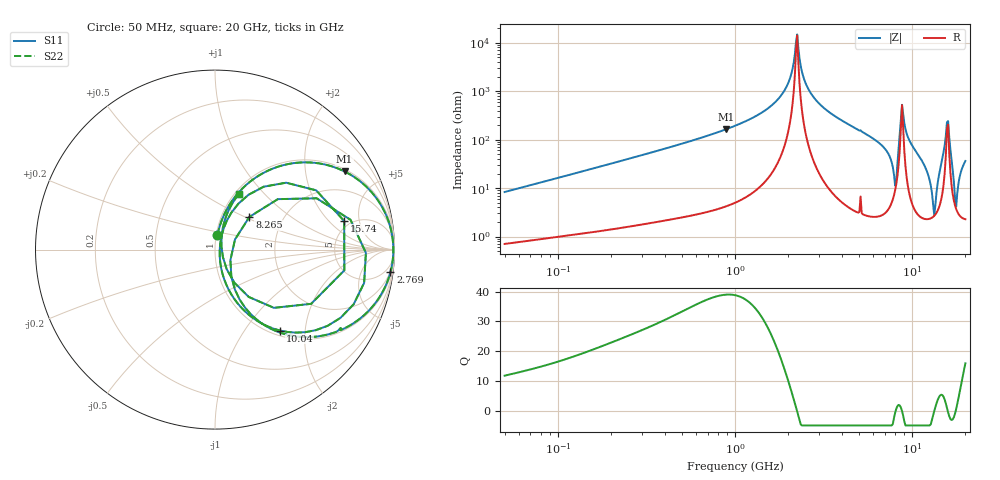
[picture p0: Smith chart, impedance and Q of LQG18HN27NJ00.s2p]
!Murata Part Number: LQG18HN27NJ00
!These Parameters are Measured in Series Mode Connection
!  o--[Z]--o
!Port1  Port2
!  o-------o
!Freq. Start=50[MHz] Stop=20[GHz], 401[Steps]
# Hz S RI R 50
!Freq.(Hz) S11(Real) S11(Imag) S21(Real) S21(Imag) S12(Real) S12(Imag) S22(Real) S22(Imag)
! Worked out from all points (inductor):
!   401 points, 50 MHz to 20 GHz, reference 50 ohm
!   read as one part in series: L = 26.1 nH near 51.52 MHz
!   highest Q = 39 at 887.1 MHz (marker M1), where L = 29.2 nH
!   self-resonance near 2.212 GHz
!   S11 on the Smith chart (normalised r, x): 50 MHz: 1.01, +0.17; 2.769 GHz: 2, -15; 8.265 GHz: 1.36, +0.53; 10.04 GHz: 1.09, -1.48; 15.74 GHz: 4.40, +3.07; 20 GHz: 1.05, +0.72
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5e7  0.0137 0.0811  0.9863 -0.0811  0.9863 -0.0811  0.0137 0.0811
1.364002e8  0.0559 0.2051  0.9441 -0.2051  0.9441 -0.2051  0.0559 0.2051
3.721004e8  0.2728 0.4288  0.7272 -0.4288  0.7272 -0.4288  0.2728 0.4288
8.870719e8  0.7217 0.4355  0.2783 -0.4355  0.2783 -0.4355  0.7217 0.4355
1e9  0.7827 0.3997  0.2173 -0.3997  0.2173 -0.3997  0.7827 0.3997
1.793498e9  0.9763 0.1272  0.0237 -0.1272  0.0237 -0.1272  0.9763 0.1272
2.021818e9  0.9898 0.0591  0.0102 -0.0591  0.0102 -0.0591  0.9898 0.0591
2.245319e9  0.9936 -0.00204  0.00638 0.00204  0.00638 0.00204  0.9936 -0.00204
2.728004e9  0.9795 -0.1178  0.0205 0.1178  0.0205 0.1178  0.9795 -0.1178
2.769174e9  0.9772 -0.1268  0.0228 0.1268  0.0228 0.1268  0.9772 -0.1268
7.442007e9  0.1972 -0.3576  0.8028 0.3576  0.8028 0.3576  0.1972 -0.3576
7.901521e9  0.0909 -0.1504  0.9091 0.1504  0.9091 0.1504  0.0909 -0.1504
8.264682e9  0.1922 0.1827  0.8078 -0.1827  0.8078 -0.1827  0.1922 0.1827
8.907419e9  0.831 -0.1852  0.169 0.1852  0.169 0.1852  0.831 -0.1852
1.004137e10  0.3632 -0.4512  0.6368 0.4512  0.6368 0.4512  0.3632 -0.4512
1.201863e10  0.0736 -0.2179  0.9264 0.2179  0.9264 0.2179  0.0736 -0.2179
1.334722e10  0.0262 -0.00238  0.9738 0.00238  0.9738 0.00238  0.0262 -0.00238
1.504638e10  0.2719 0.3506  0.7281 -0.3506  0.7281 -0.3506  0.2719 0.3506
1.573793e10  0.7199 0.1592  0.2801 -0.1592  0.2801 -0.1592  0.7199 0.1592
1.646126e10  0.3285 -0.3245  0.6715 0.3245  0.6715 0.3245  0.3285 -0.3245
1.774144e10  0.036 0.0176  0.964 -0.0176  0.964 -0.0176  0.036 0.0176
2e10  0.1311 0.3075  0.8689 -0.3075  0.8689 -0.3075  0.1311 0.3075
